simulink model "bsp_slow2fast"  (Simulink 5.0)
settings: Solver=FixedStepDiscrete  StartTime=0.0  StopTime=20.0  RelTol=1e-3
libraries: simulink x1

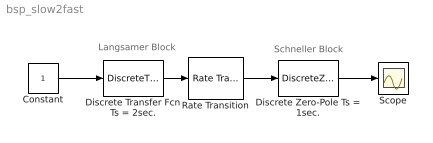
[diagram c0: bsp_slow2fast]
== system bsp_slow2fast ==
  note: Langsamer Block
  note: Schneller Block
  Constant : Constant
  Discrete Transfer Fcn Ts = 2sec. : DiscreteTransferFcn  SampleTime=2
  Discrete Zero-Pole Ts = 1sec. : DiscreteZeroPole  Poles=[0 0.5]  Gain=1
  Rate Transition : simulink/Signal Attributes/Rate Transition  DataIntegrity=on  DeterministicTransfer=on  TransitionType=Slow to fast  InitCond=0
  Scope : Scope
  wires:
  Constant/1 -> Discrete Transfer Fcn Ts = 2sec./1
  Discrete Zero-Pole Ts = 1sec./1 -> Scope/1
  Discrete Transfer Fcn Ts = 2sec./1 -> Rate Transition/1
  Rate Transition/1 -> Discrete Zero-Pole Ts = 1sec./1
